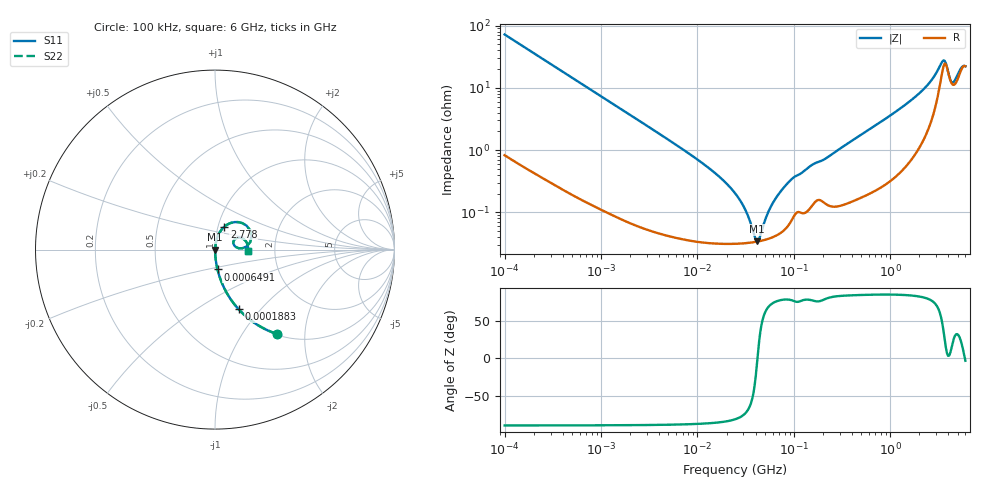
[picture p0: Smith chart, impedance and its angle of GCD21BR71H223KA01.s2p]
!Murata Part Number: GCD21BR71H223KA01
!These Parameters are Measured in Series Mode Connection
!Data Generated on Jan 08, 2026
!  o--ll--o
!Port1  Port2
!  o------o
!Operation Temp=25[degC], DC Bias Voltage=0[V]
!Freq. Start=100[kHz] Stop=6[GHz] 401[Steps]
# Hz S RI R 50
!Freq.(Hz) S11(Real) S11(Imag) S21(Real) S21(Imag) S12(Real) S12(Imag) S22(Real) S22(Imag)
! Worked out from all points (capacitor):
!   401 points, 100 kHz to 6 GHz, reference 50 ohm
!   read as one part in series: C = 22 nF near 105.7 kHz
!   lowest |Z| = 34 mohm at 41.31 MHz (marker M1)
!   series resonance near 41.88 MHz, so ESL is about 660 pH
!   S11 on the Smith chart (normalised r, x): 100 kHz: 1.02, -1.44; 188.3 kHz: 1.01, -0.77; 649.1 kHz: 1.00, -0.23; 2.778 GHz: 1.07, +0.28; 6 GHz: 1.44, -0.02
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100000  0.3438 -0.4693  0.6562 0.4693  0.6562 0.4693  0.3438 -0.4693
188254  0.1319 -0.3325  0.8681 0.3325  0.8681 0.3325  0.1319 -0.3325
631452  0.0147 -0.1138  0.9853 0.1138  0.9853 0.1138  0.0147 -0.1138
649061  0.014 -0.1108  0.986 0.1108  0.986 0.1108  0.014 -0.1108
3987316  0.000794 -0.0184  0.9992 0.0184  0.9992 0.0184  0.000794 -0.0184
1.374747e7  0.00034 -0.00484  0.9997 0.00484  0.9997 0.00484  0.00034 -0.00484
2.517799e7  0.000315 -0.00189  0.9997 0.00189  0.9997 0.00189  0.000315 -0.00189
3.137502e7  0.000319 -0.00105  0.9997 0.00105  0.9997 0.00105  0.000319 -0.00105
4.130835e7  0.000336 -4.92e-05  0.9997 4.92e-05  0.9997 4.92e-05  0.000336 -4.92e-05
4.36444e7  0.000342 0.000148  0.9997 -0.000148  0.9997 -0.000148  0.000342 0.000148
5.590324e7  0.000381 0.00105  0.9996 -0.00105  0.9996 -0.00105  0.000381 0.00105
6.966265e7  0.000448 0.00192  0.9996 -0.00192  0.9996 -0.00192  0.000448 0.00192
9.690463e7  0.0008 0.00342  0.9992 -0.00342  0.9992 -0.00342  0.0008 0.00342
1.546735e8  0.00131 0.00563  0.9987 -0.00563  0.9987 -0.00563  0.00131 0.00563
9.76689e8  0.00429 0.0347  0.9957 -0.0347  0.9957 -0.0347  0.00429 0.0347
1.889928e9  0.0148 0.0734  0.9852 -0.0734  0.9852 -0.0734  0.0148 0.0734
2.77767e9  0.0525 0.1279  0.9475 -0.1279  0.9475 -0.1279  0.0525 0.1279
3.557862e9  0.1958 0.1081  0.8042 -0.1081  0.8042 -0.1081  0.1958 0.1081
3.971646e9  0.1527 0.00746  0.8473 -0.00746  0.8473 -0.00746  0.1527 0.00746
4.433555e9  0.1025 0.0347  0.8975 -0.0347  0.8975 -0.0347  0.1025 0.0347
5.087202e9  0.135 0.0669  0.865 -0.0669  0.865 -0.0669  0.135 0.0669
6e9  0.1818 -0.00832  0.8182 0.00832  0.8182 0.00832  0.1818 -0.00832
